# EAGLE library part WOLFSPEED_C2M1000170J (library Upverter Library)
N-Channel 5.3A (Tc) 78W (Tc) Surface Mount D2PAK (7-Lead)
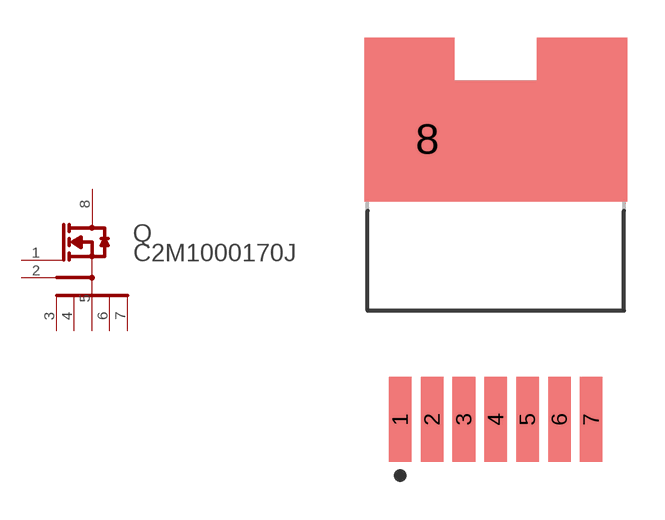
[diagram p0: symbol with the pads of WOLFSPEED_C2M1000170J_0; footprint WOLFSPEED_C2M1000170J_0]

Designator prefix Q

## WOLFSPEED_C2M1000170JWOLFSPEED_C2M1000170J_0_0 (MF: Wolfspeed; MPN: C2M1000170J; automotive: No; centroid_not_specified: Yes; continuous_drain_current: 5.6A; datasheet: https://assets.wolfspeed.com/uploads/2020/12/C2M1000170J.pdf; depletion_mode: False; device_class_L1: Discrete Semiconductors; device_class_L2: Transistors; device_class_L3: MOSFETs; digikey_description: SICFET N-CH 1700V 5.3A D2PAK; digikey_part_number: C2M1000170J-ND; drain_to_source_breakdown_voltage: 1700V; drain_to_source_resistance: 0.8Ω; drain_to_source_voltage: 1700V; footprint_variant_name_0: Recommended_Land_Pattern; gate_charge_at_vgs: 13nC @ 20V; gate_to_source_voltage: 20V; height: 4.82mm; input_capacitace_at_vds: 215pF @ 1000V; lead_free: Yes; max_junction_temp: +150°C; mfg_package_ident: TO-263-7; mfg_package_ident_component_id: d2de6d38281de76c; mfg_package_ident_date: 0; mfg_package_ident_rev: 0; mouser_part_number: 941-C2M1000170J; number_of_N_channels: 1; number_of_channels: 1; package: TO-263-7; power_dissipation: 60W; prefix: Q; pulse_drain_current: 15A; reverse_recovery_charge: 31nC; reverse_recovery_time: 15ns; rohs: Yes; rthja_max: 40°C/W; standoff_height: 0mm; technology: SiC; temperature_range_high: +150°C; temperature_range_low: -55°C; threshold_vgs_max: 4V; threshold_vgs_min: 2V; transconductance: 1.04S; turn_off_delay_time: 12.6ns; turn_on_delay_time: 4.2ns; typ_forward_diode_voltage: 3.8V; verification_version: 0.0.0.3)  [WOLFSPEED_C2M1000170J_0]
1  GATE  pas
2  DRIVER_SOURCE  pas
3  1_POWER_SOURCE  pas
4  2_POWER_SOURCE  pas
5  3_POWER_SOURCE  pas
6  4_POWER_SOURCE  pas
7  5_POWER_SOURCE  pas
8  DRAIN  pas

## Footprint WOLFSPEED_C2M1000170J_0 (pad centres in mm)
N-Channel 5.3A (Tc) 78W (Tc) Surface Mount D2PAK (7-Lead)
smd 0.9 x 3.4: 1 -3.81,-6.764; 2 -2.54,-6.764; 3 -1.27,-6.764; 4 0,-6.764; 5 1.27,-6.764; 6 2.54,-6.764; 7 3.81,-6.764
smd 4.505 x 4.505: 8 -2.737,4.429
